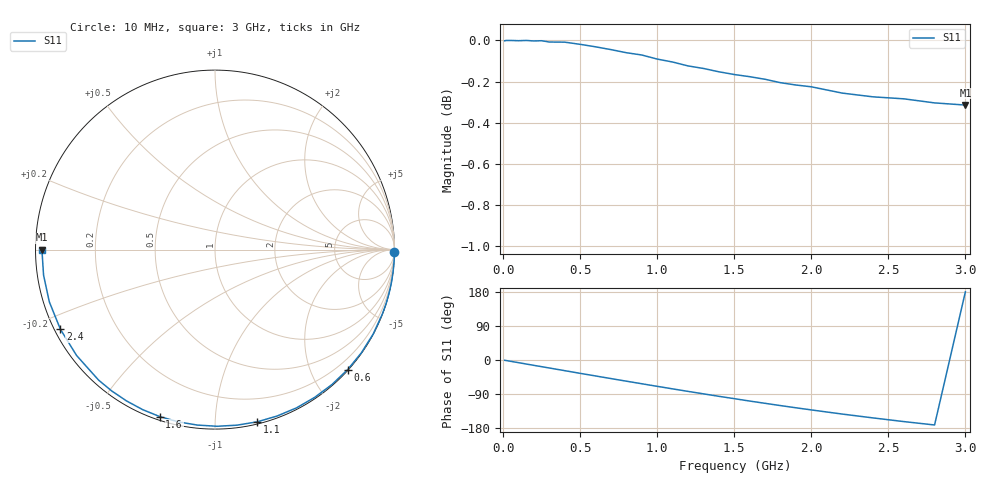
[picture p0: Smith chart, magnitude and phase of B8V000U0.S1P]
! SIEMENS Discrete & RF Semiconductors
! BBY53-03W
! Si Tuning Diode in SOD323
! VR = 0 V
! S-Parameters:  May  1997
# GHz  S  MA  R  50
!  f  S11
! GHz  MAG  ANG
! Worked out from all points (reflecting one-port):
!   30 points, 10 MHz to 3 GHz, reference 50 ohm
!   lowest |S11| = -0.3 dB at 3 GHz (marker M1), VSWR 55.31, Z = 0.904 + j3.06e-15 ohm
!   phase of S11 starts at -1 deg and turns -179 deg over the sweep
!   S11 on the Smith chart (normalised r, x): 10 MHz: open; 600 MHz: 0.01, -2.60; 1.1 GHz: 0.02, -1.28; 1.6 GHz: 0.02, -0.72; 2.4 GHz: 0.02, -0.24; 3 GHz: 0.02, +0.00
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0.01  0.9998 -0.7
0.1  0.9999 -7.0
0.15  1 -10.6
0.2  0.9997 -14.1
0.25  0.9998 -17.6
0.3  0.9991 -21.1
0.4  0.999 -28.1
0.5  0.9978 -35.2
0.6  0.9964 -42.1
0.7  0.9949 -49.0
0.8  0.9931 -55.9
0.9  0.9919 -62.7
1  0.9896 -69.5
1.1  0.988 -76.2
1.2  0.9858 -82.8
1.3  0.9845 -89.3
1.4  0.9826 -95.8
1.5  0.9811 -102.0
1.6  0.9799 -108.3
1.7  0.9785 -114.3
1.8  0.9766 -120.3
1.9  0.9754 -126.1
2  0.9744 -131.7
2.2  0.971 -142.6
2.4  0.9689 -152.8
2.6  0.9679 -162.5
2.8  0.9657 -171.5
3  0.9645 180.0
